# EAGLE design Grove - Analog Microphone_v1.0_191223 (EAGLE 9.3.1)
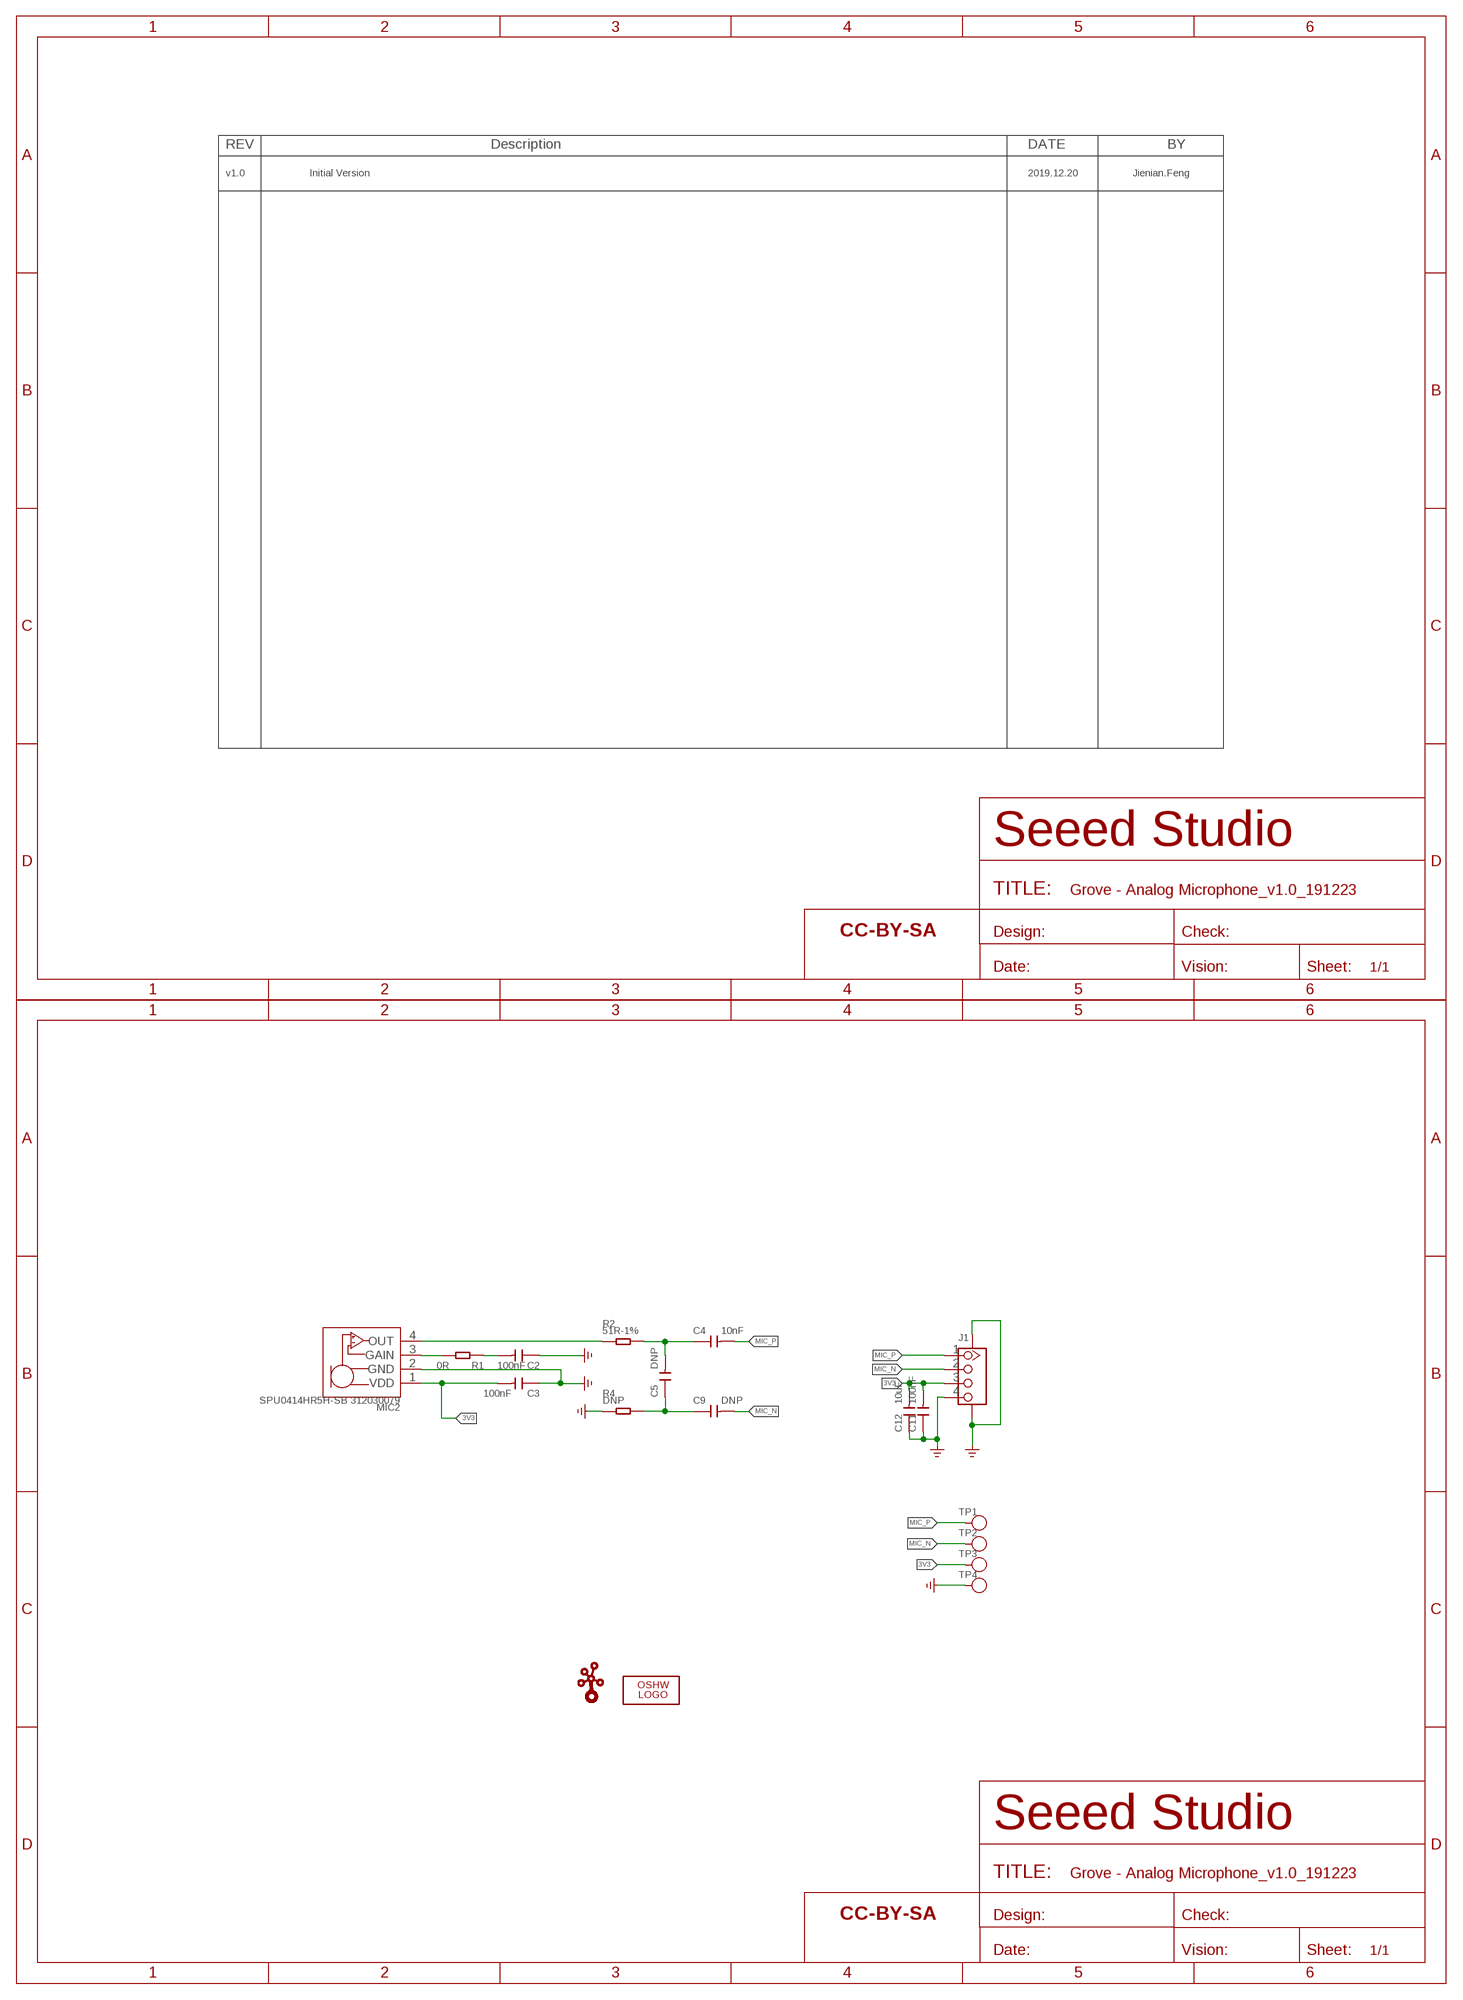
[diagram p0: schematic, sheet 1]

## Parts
C2  100nF  CAP-0603  [C0603]
C3  100nF  CAP-0603  [C0603]
C4  10nF  CAP-0603  [C0603]
C5  DNP  CAP-0603  [C0603]
C9  DNP  CAP-0603  [C0603]
C11  100nF  CAP-0603  [C0603]
C12  10uF  CAP-0603  [C0603]
FR1  SEEEDSTUDIO-OPEN-SCH-FRAME  [SEEEDSTUDIO-PCB-FRAME]
FR2  SEEEDSTUDIO-OPEN-SCH-FRAME  [SEEEDSTUDIO-PCB-FRAME]
J1  GROVE-CONNECTOR-SMD-320110030  [HW4-SMD-2.0]
LOGO1  LOGO-OSHW-FILLX0200-NT  [OSHW_FILLX200_NOTEXT]
MIC2  SPU0414HR5H-SB 312030079  MICROPHONE-SPU0414HR5H-SB-312030079  [MIC4P-1.7-3.76X2.95X1.1MM]
R1  0R  RES-0603  [R0603]
R2  51R-1%  RES-0603  [R0603]
R4  DNP  RES-0603  [R0603]
TP1  TEST-POINT'4545'  [TP-D45MIL]
TP2  TEST-POINT'4545'  [TP-D45MIL]
TP3  TEST-POINT'4545'  [TP-D45MIL]
TP4  TEST-POINT'4545'  [TP-D45MIL]
U$4  LOGO-GROVE  [GROVE-SILK-BIG]

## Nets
3V3: C3.2 C11.2 C12.2 J1.3 MIC2.1(VDD) TP3.T
GND: C2.1 C3.1 C11.1 C12.1 J1.4 J1.SS1 J1.SS2 MIC2.2(GND) R4.1 TP4.T ; supply symbol labelled GND_POWER
MIC_N: C9.2 J1.2 TP2.T
MIC_P: C4.2 J1.1 TP1.T
N$1: MIC2.3(GAIN) R1.2
N$2: C2.2 R1.1
N$3: C4.1 C5.2 R2.2
N$4: C5.1 C9.1 R4.2
SIG1: MIC2.4(OUT) R2.1

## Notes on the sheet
- v1.0 | Initial Version | 2019.12.20 | Jienian.Feng

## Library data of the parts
C2-C5 C9 C11 C12 = Discrete-new:CAP: Ceramic Capacitors
FR1 FR2 = moudle-new:SEEEDSTUDIO-OPEN-SCH-FRAME
J1 = Connector-new:GROVE-CONNECTOR-SMD
LOGO1 = logo:LOGO-OSHW-FILL; PARTNO: DNP
MIC2 = Discrete-new:MICROPHONE-SPU0414HR5H-SB
R1 R2 R4 = Discrete-new:RES
TP1-TP4 = Discrete-new:TEST-POINT; PARTNO: DNP
U$4 = logo:LOGO-GROVE; PARTNO: DNP

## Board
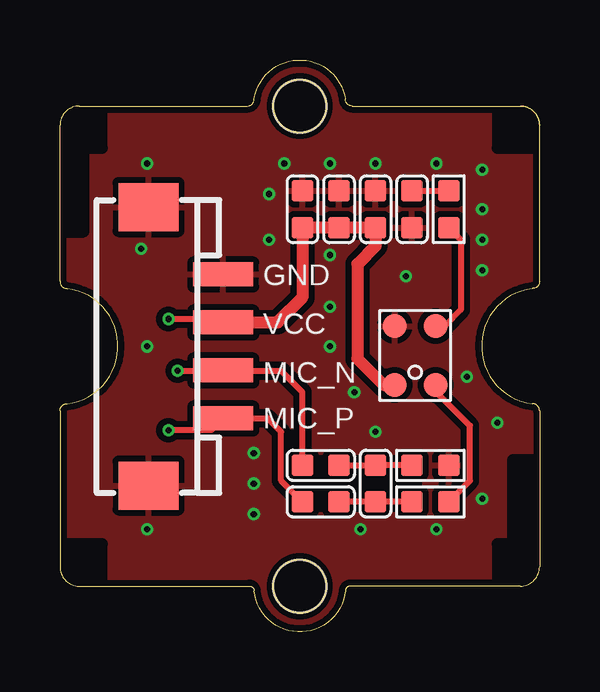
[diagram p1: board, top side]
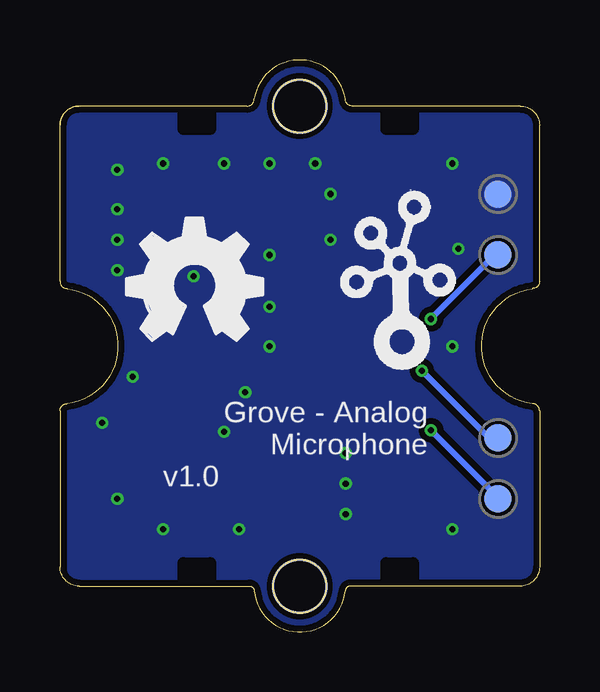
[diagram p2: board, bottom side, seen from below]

Size 20 x 23.83 mm. Coordinates in mm from the lower left corner, seen from the top.
Copper layers (1*16): Top 0.035mm / dielectric 1.5mm / Bottom 0.035mm
Design rules "SeeedStudio_2layer_DRU_no_angle_20140221": minimum track width 1mil, minimum drill 10mil, track to track 6mil, track to pad 6mil, pad to pad 6mil, via to via 6mil, smd to smd 0mil, copper to edge 10mil, drill to drill 10mil, minimum pad ring 4mil, minimum via ring 4mil, stop-mask expansion 2mil, vias tented up to drill 25mil, thermal gap 10mil

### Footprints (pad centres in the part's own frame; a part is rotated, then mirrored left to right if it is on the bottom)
C0603 = smd 0.889 x 0.889: 1 -0.762,0; 2 0.762,0
HW4-SMD-2.0 = smd 1 x 2.5: 1 -3,0; 2 -1,0; 3 1,0; 4 3,0 | smd 2 x 2.5: SS1 -5.8,3.123; SS2 5.8,3.123
MIC4P-1.7-3.76X2.95X1.1MM = smd 1 x 1: 1 0.85,1.23; 2 0.85,-1.23; 3 -0.85,-1.23; 4 -0.85,1.23
R0603 = smd 0.889 x 0.889: 1 -0.762,0; 2 0.762,0
TP-D45MIL = smd 1.143 x 1.143: T 0,0
GROVE-1X1-TEST-PLATFORM-TOP = hole 2.2: 9.987,0.013; -10.013,0.013

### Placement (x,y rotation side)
C2  14.69,17.61 90 top
C3  13.16,17.61 270 top
C4  10.88,5.42 180 top
C5  13.16,6.18 270 top
C9  10.88,6.94 180 top
C11  11.64,17.61 270 top
C12  10.11,17.61 270 top
FR1  not placed on the board
FR2  not placed on the board
J1  6.81,11.9 90 top
LOGO1  17.23,12.15 0 bottom
MIC2  14.81,11.51 180 top
R1  16.21,17.61 270 top
R2  15.45,5.42 180 top
R4  15.45,6.94 180 top
TP1  1.73,5.55 90 bottom
TP2  1.73,8.09 90 bottom
TP3  1.73,15.71 90 bottom
TP4  1.73,18.25 90 bottom
U$2  [GROVE-1X1-TEST-PLATFORM-TOP]  9.99,11.9 270 top
U$4  5.8,11.9 0 bottom

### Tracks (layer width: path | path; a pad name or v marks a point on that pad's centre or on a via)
3V3  (via drill 0.25 pad 0.51)
  Top 0.254: v4.53,13.04 6.67,13.04 J1.3
  Top 0.508: J1.3 9.08,12.9 10.11,13.93 C12.2 C11.2 C3.2 13.16,16.09 12.4,15.32 12.4,11.39 13.5,10.28 MIC2.1
  Bottom 0.254: TP3.T 1.86,15.71 v4.53,13.04
GND  (via drill 0.25 pad 0.51)
  other vias: 17.61,19.26 11.26,13.55 17.61,16.34 14.43,14.82 8.08,6.18 12.27,9.99 13.16,8.34 11.26,15.71 11.26,11.9 8.08,7.45 8.08,4.91 15.7,4.28 12.53,4.28 18.24,8.72 17.61,5.55 17.61,17.61 17.61,15.07 13.16,19.52 11.26,19.52 9.35,19.52 15.7,19.52 8.72,16.34 3.38,15.96 3.64,19.52 3.64,11.9 3.64,4.28 8.72,18.25 16.97,10.63
  pour Top (isolate 0.254): -0.81,24.6 20.78,24.6 20.78,-0.8 -0.81,-0.8
  pour Bottom (isolate 0.254): -0.81,24.6 20.78,24.6 20.78,-0.8 -0.81,-0.8
MIC_N  (via drill 0.25 pad 0.51)
  Top 0.254: v4.91,10.88 6.8,10.88 | 6.8,10.88 J1.2 | 10.04,6.94 C9.2 10.11,9.99 9.23,10.88 6.8,10.88
  Bottom 0.254: TP2.T 2.11,8.09 v4.91,10.88
MIC_P  (via drill 0.25 pad 0.51)
  Top 0.254: v4.53,8.4 6.32,8.4 J1.1 6.8,8.91 8.65,8.91 9.23,8.34 9.23,6.31 10.04,5.49 10.04,5.42 C4.2
  Bottom 0.254: TP1.T 1.73,5.61 v4.53,8.4
N$1
  Top 0.254: R1.2 16.72,16.34 16.72,13.42 16.04,12.74 MIC2.3
N$2
  Top 0.254: C2.2 R1.1
N$3
  Top 0.254: R2.2 C5.2 C4.1
N$4
  Top 0.254: C9.1 C5.1 R4.2
SIG1
  Top 0.254: R2.1 17.1,6.31 17.1,8.59 15.66,10.03 MIC2.4

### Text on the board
tPlace: GND | VCC | MIC_N | MIC_P
bNames: Grove - Analog / Microphone | v1.0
